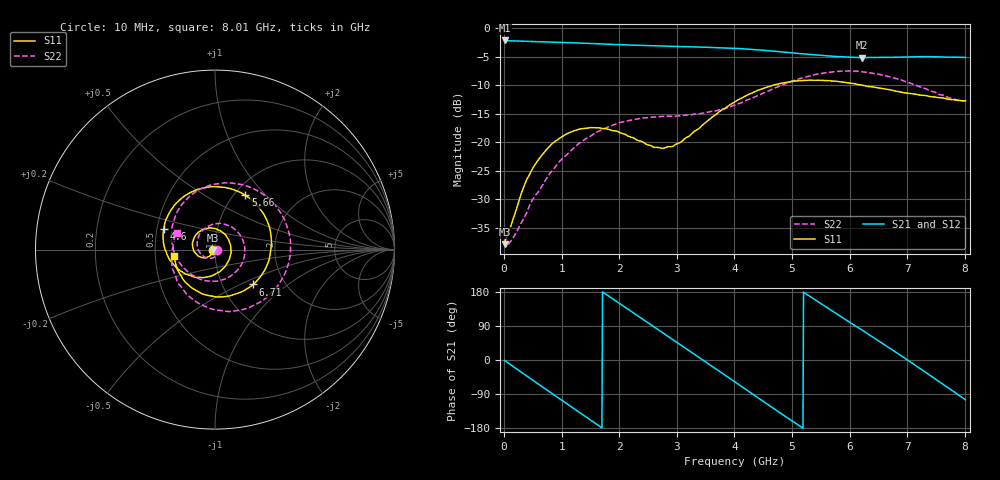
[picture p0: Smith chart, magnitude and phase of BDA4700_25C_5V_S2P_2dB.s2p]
!Agilent Technologies,E5071B,MY42404982,A.09.10
!Date: Mon Oct 20 13:26:54 2025
!Data & Calibration Information:
!Freq	S11:SOLT2(ON)	S21:SOLT2(ON)	S12:SOLT2(ON)	S22:SOLT2(ON)
# Hz S RI R 50
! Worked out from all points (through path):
!   801 points, 10 MHz to 8.01 GHz, reference 50 ohm
!   highest |S21| = -2.11 dB at 10 MHz (marker M1); lowest = -5.1 dB at 6.22 GHz (marker M2)
!   group delay of S21, straight-line fit = 285 ps
!   lowest |S11| = -38.0 dB at 10 MHz (marker M3), VSWR 1.03, Z = 48.8 - j0.186 ohm
!   |S11| at or under -10 dB: start of sweep to 4.665 GHz; 6.23 GHz to end of sweep
!   |S22| runs from -38.3 to -7.5 dB; largest |S21 - S12| = 0.0062
!   S11 on the Smith chart (normalised r, x): 10 MHz: 0.98, -0.00; 4.6 GHz: 0.54, +0.14; 5.66 GHz: 1.13, +0.77; 6.71 GHz: 1.40, -0.59; 8.01 GHz: 0.63, -0.05
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1e7  -0.0125 -0.00191  0.7838 -0.0169  0.7838 -0.0178  0.0134 -0.00158
3.3e8  -0.0243 -0.0306  0.6294 -0.447  0.6292 -0.448  0.0152 -0.0142
7.2e8  -0.0712 -0.0446  0.1765 -0.7406  0.1765 -0.7408  -0.00993 -0.0453
1.02e9  -0.1115 -0.0171  -0.2336 -0.7156  -0.2344 -0.7157  -0.0595 -0.0406
1.35e9  -0.124 0.0427  -0.5905 -0.4498  -0.591 -0.4501  -0.0989 0.0217
1.64e9  -0.0946 0.0948  -0.7275 -0.09  -0.7276 -0.09  -0.0772 0.098
1.93e9  -0.037 0.1201  -0.6642 0.283  -0.6648 0.2834  0.00304 0.1436
2.32e9  0.0445 0.0936  -0.319 0.6346  -0.319 0.635  0.1274 0.0974
2.68e9  0.0865 0.0239  0.1254 0.6907  0.1259 0.6905  0.1651 -0.0294
3.36e9  0.0164 -0.1282  0.6771 0.1142  0.6776 0.1138  -0.0129 -0.1764
3.67e9  -0.0773 -0.1555  0.6261 -0.2604  0.6261 -0.2619  -0.1171 -0.1473
4.01e9  -0.1939 -0.1176  0.3535 -0.5664  0.3537 -0.566  -0.2014 -0.0669
4.6e9  -0.2854 0.1162  -0.3136 -0.5539  -0.3136 -0.5543  -0.2258 0.1697
4.98e9  -0.1883 0.2841  -0.569 -0.2228  -0.5706 -0.2242  -0.1012 0.3262
5.35e9  0.000532 0.3507  -0.5656 0.1622  -0.5662 0.161  0.1207 0.3667
5.66e9  0.1691 0.3022  -0.3916 0.4159  -0.3915 0.4165  0.3051 0.2775
6.22e9  0.3146 0.0377  0.1092 0.5428  0.1154 0.543  0.4069 -0.0856
6.68e9  0.2241 -0.1843  0.4685 0.3016  0.4697 0.3009  0.2086 -0.314
6.71e9  0.2134 -0.1943  0.4838 0.2767  0.4852 0.2753  0.1901 -0.3232
7.27e9  -0.0439 -0.2543  0.5015 -0.2601  0.5002 -0.2609  -0.1354 -0.2687
7.65e9  -0.1781 -0.1656  0.2187 -0.5162  0.2168 -0.5175  -0.2401 -0.0886
8.01e9  -0.2283 -0.0372  -0.1432 -0.5364  -0.1425 -0.537  -0.2099 0.0947
